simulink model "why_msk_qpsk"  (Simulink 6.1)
settings: Solver=ode45  StartTime=0.0  StopTime=inf  RelTol=1e-3
libraries: commsink2 x4, commchan2 x2, commrandsrc2 x2, commdigbbndcpm2 x1, commdigbbndpm2 x1, commfilt2 x1

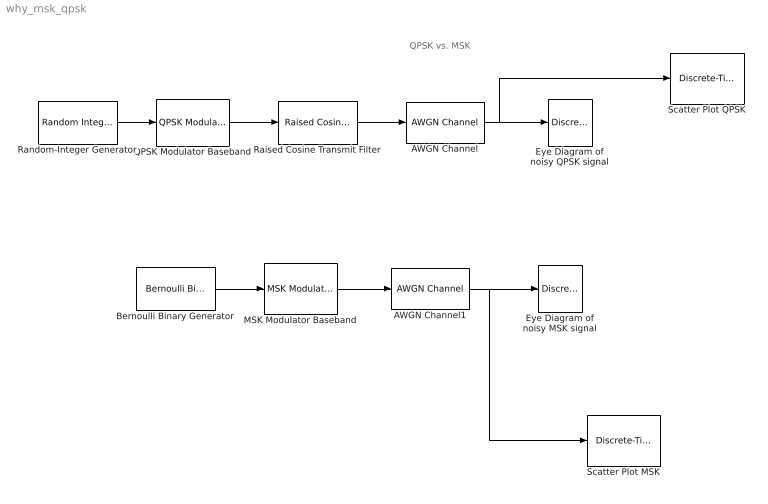
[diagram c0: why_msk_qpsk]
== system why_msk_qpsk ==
  note: QPSK vs. MSK
  AWGN Channel : commchan2/AWGN Channel  seed=1237  noiseMode="Signal to noise ratio  (SNR)"  EbNodB=10  EsNodB=10  SNRdB=30  bitsPerSym=1  Ps=1  Tsym=1  variance=1
  AWGN Channel1 : commchan2/AWGN Channel  seed=1237  noiseMode="Signal to noise ratio  (SNR)"  EbNodB=10  EsNodB=10  SNRdB=30  bitsPerSym=1  Ps=1  Tsym=1  variance=1
  Bernoulli Binary Generator : commrandsrc2/Bernoulli Binary Generator  P=0.5  seed=61  Ts=0.5  frameBased=off  sampPerFrame=1  orient=off
  Eye Diagram of noisy MSK signal : commsink2/Discrete-Time Eye Diagram Scope  Tag=EyeDiagram  sampPerSymb=8  offsetEye=4  symbPerTrace=4  numTraces=40  numNewFrames=10  LineStyles=-  LineColors=m  dupPoints=on  fading=on  render=on  AxisGrid=on  yMin=-1.5  yMax=1.5  inphaseLabel=In-phase Amplitude  quadratureLabel=Quadrature Amplitude  openScopeAtSimStart=on  dispDiagram=In-phase and Quadrature  FrameNumber=off  FigPos=[512 225 358 412]  figTitle=Eye Diagram  block_type_=eye  numLinesMax=8
  Eye Diagram of noisy QPSK signal : commsink2/Discrete-Time Eye Diagram Scope  Tag=EyeDiagram  sampPerSymb=8  offsetEye=0  symbPerTrace=2  numTraces=40  numNewFrames=10  LineStyles=-  LineColors=b  dupPoints=on  fading=on  render=on  AxisGrid=on  yMin=-1.5  yMax=1.5  inphaseLabel=In-phase Amplitude  quadratureLabel=Quadrature Amplitude  openScopeAtSimStart=on  dispDiagram=In-phase and Quadrature  FrameNumber=off  FigPos=[51 225 358 412]  figTitle=Eye Diagram  block_type_=eye  numLinesMax=8
  MSK Modulator Baseband : commdigbbndcpm2/MSK Modulator Baseband  inputType=Bit  phaseOffset=0  samplesPerSymbol=8
  QPSK Modulator Baseband : commdigbbndpm2/QPSK Modulator Baseband  InType=Integer  Enc=Binary  Ph=pi/4  numSamp=1
  Raised Cosine Transmit Filter : commfilt2/Raised Cosine Transmit Filter  filtType=Normal  D=1  R=0.3  sampMode=Sample-based  N=8  checkGain=Normalized  filterGain=1  checkCoeff=off  variableName=rcTxFilt  launchFVT=off
  Random-Integer Generator : commrandsrc2/Random Integer Generator  mul=4  seed=[12345]  Ts=1  frameBased=off  sampPerFrame=50  orient=off
  Scatter Plot MSK : commsink2/Discrete-Time Scatter Plot Scope  Tag=ScatterPlot  sampPerSymb=1  offsetEye=0  numTraces=40  numNewFrames=10  LineMarkers=.  LineColors=b  fading=on  render=on  AxisGrid=on  xMin=-1.5  xMax=1.5  yMin=-1.5  yMax=1.5  inphaseLabel=In-phase Amplitude  quadratureLabel=Quadrature Amplitude  openScopeAtSimStart=on  FrameNumber=off  FigPos=[232 106 560 560]  figTitle=Scatter Plot  numLinesMax=8  block_type_=scatter
  Scatter Plot QPSK : commsink2/Discrete-Time Scatter Plot Scope  Tag=ScatterPlot  sampPerSymb=1  offsetEye=0  numTraces=40  numNewFrames=10  LineMarkers=.  LineColors=b  fading=on  render=on  AxisGrid=on  xMin=-1.5  xMax=1.5  yMin=-1.5  yMax=1.5  inphaseLabel=In-phase Amplitude  quadratureLabel=Quadrature Amplitude  openScopeAtSimStart=on  FrameNumber=off  FigPos=[232 106 560 560]  figTitle=Scatter Plot  numLinesMax=8  block_type_=scatter
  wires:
  Bernoulli Binary Generator/1 -> MSK Modulator Baseband/1
  MSK Modulator Baseband/1 -> AWGN Channel1/1
  AWGN Channel1/1 -> Eye Diagram of noisy MSK signal/1, Scatter Plot MSK/1
  QPSK Modulator Baseband/1 -> Raised Cosine Transmit Filter/1
  AWGN Channel/1 -> Eye Diagram of noisy QPSK signal/1, Scatter Plot QPSK/1
  Random-Integer Generator/1 -> QPSK Modulator Baseband/1
  Raised Cosine Transmit Filter/1 -> AWGN Channel/1
